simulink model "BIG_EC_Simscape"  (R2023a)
settings: Solver=VariableStepAuto  StartTime=0.0  StopTime=10.0  RelTol=1e-3
libraries: fl_lib x18

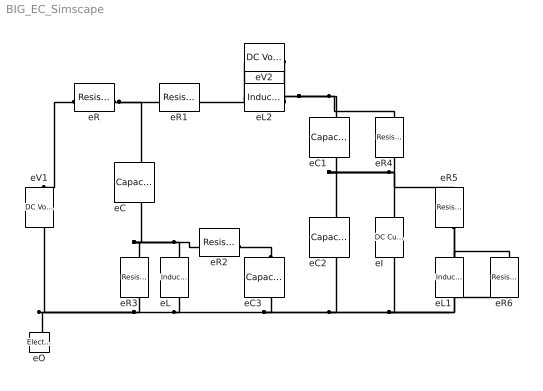
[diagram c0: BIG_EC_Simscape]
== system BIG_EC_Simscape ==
  eC{,1..3} (4 alike) : fl_lib/Electrical/Electrical Elements/Capacitor  c=1e-6 F  r=1e-6 Ohm  g=0 1/Ohm  i_specify=off  i_priority=None  i=0 A  i_nominal_specify=off  i_nominal_unit=A  i_nominal_value=1  v_specify=off  v_priority=None  v=0 V  v_nominal_specify=off  v_nominal_unit=V  v_nominal_value=1  vc_specify=off  vc_priority=High  vc=0 V  vc_nominal_specify=off  vc_nominal_unit=V  vc_nominal_value=1
  eI : fl_lib/Electrical/Electrical Sources/DC Current Source  i0=1 A
  eL : fl_lib/Electrical/Electrical Elements/Inductor  l=1e-6 H  r=0 Ohm  g=1e-9 1/Ohm  i_specify=off  i_priority=None  i=0 A  i_nominal_specify=off  i_nominal_unit=A  i_nominal_value=1  v_specify=off  v_priority=None  v=0 V  v_nominal_specify=off  v_nominal_unit=V  v_nominal_value=1  i_L_specify=off  i_L_priority=High  i_L=0 A  i_L_nominal_specify=off  i_L_nominal_unit=A  i_L_nominal_value=1
  eL1 : fl_lib/Electrical/Electrical Elements/Inductor  l=1e-6 H  r=0 Ohm  g=1e-9 1/Ohm  i_specify=off  i_priority=None  i=0 A  i_nominal_specify=off  i_nominal_unit=A  i_nominal_value=1  v_specify=off  v_priority=None  v=0 V  v_nominal_specify=off  v_nominal_unit=V  v_nominal_value=1  i_L_specify=off  i_L_priority=High  i_L=0 A  i_L_nominal_specify=off  i_L_nominal_unit=A  i_L_nominal_value=1
  eL2 : fl_lib/Electrical/Electrical Elements/Inductor  l=1e-6 H  r=0 Ohm  g=1e-9 1/Ohm  i_specify=off  i_priority=None  i=0 A  i_nominal_specify=off  i_nominal_unit=A  i_nominal_value=1  v_specify=off  v_priority=None  v=0 V  v_nominal_specify=off  v_nominal_unit=V  v_nominal_value=1  i_L_specify=off  i_L_priority=High  i_L=0 A  i_L_nominal_specify=off  i_L_nominal_unit=A  i_L_nominal_value=1
  eO : fl_lib/Electrical/Electrical Elements/Electrical Reference
  eR{,1..6} (7 alike) : fl_lib/Electrical/Electrical Elements/Resistor  R=1 Ohm  i_specify=off  i_priority=None  i=0 A  i_nominal_specify=off  i_nominal_unit=A  i_nominal_value=1  v_specify=off  v_priority=None  v=0 V  v_nominal_specify=off  v_nominal_unit=V  v_nominal_value=1
  eV1 : fl_lib/Electrical/Electrical Sources/DC Voltage Source  v0=1 V
  eV2 : fl_lib/Electrical/Electrical Sources/DC Voltage Source  v0=1 V
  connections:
  eV1/RConn1 -- eO/LConn1 -- eR3/RConn1 -- eL/RConn1 -- eI/RConn1 -- eL1/RConn1 -- eR6/RConn1 -- eC2/RConn1 -- eC3/RConn1
  eL/LConn1 -- eR2/LConn1 -- eC/RConn1 -- eR3/LConn1
  eC3/LConn1 -- eR2/RConn1
  eR/LConn1 -- eV1/LConn1
  eR/RConn1 -- eC/LConn1 -- eR1/LConn1
  eV2/LConn1 -- eL2/LConn1 -- eR1/RConn1
  eC1/LConn1 -- eR4/LConn1 -- eL2/RConn1 -- eV2/RConn1
  eI/LConn1 -- eR5/LConn1 -- eR4/RConn1 -- eC2/LConn1 -- eC1/RConn1
  eR5/RConn1 -- eL1/LConn1 -- eR6/LConn1
